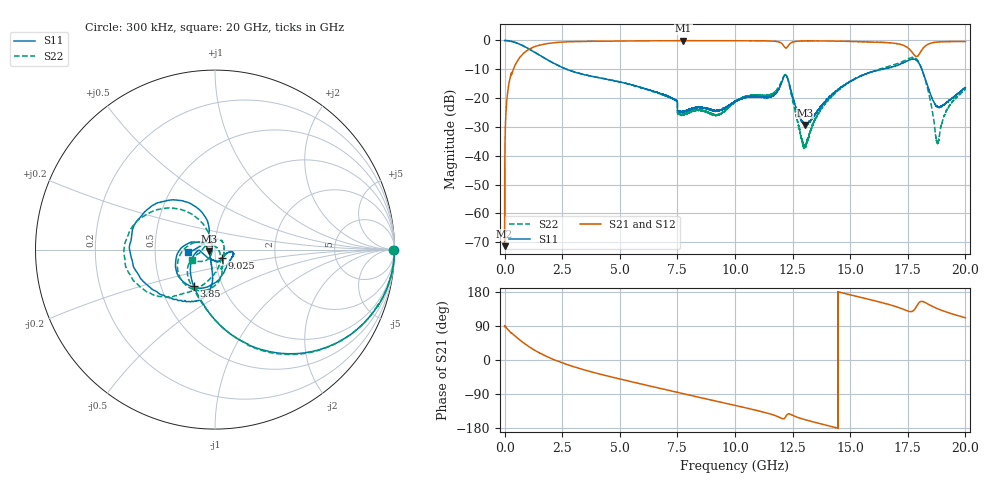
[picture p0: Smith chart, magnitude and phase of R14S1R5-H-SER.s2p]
!{R14S1R5}
!Johanson Technology Inc.
!www.johansontechnology.com
!Test Board Conditions:
!Substrate Type  RO4350B
!Substrate Thickness  20 mil
!Substrate Dk  3.66
!TL Type: GCPW
!TL Trace Width  36 mil
!TL Gap  12 mil
!Electrode orientation  Horizontal
!DUT TOPOLOGY	SERIES
!Mounting Pad LxW  26x36 mil
! Created Wed Nov 25 17:33:21 2020
! 2 Port Network Data from SP1.SP block
! freq  magS11  angS11  magS21  angS21  magS12  angS12  magS22  angS22
# khz S ma R 50
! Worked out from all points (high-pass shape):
!   20001 points, 300 kHz to 20 GHz, reference 50 ohm
!   highest |S21| = -0.06 dB at 7.757 GHz (marker M1); lowest = -71.4 dB at 300 kHz (marker M2)
!   |S21| within 3 dB of the highest: 1.064 GHz to 17.58 GHz (16.51 GHz wide, 177 % of centre); 18.13 GHz to end of sweep
!   lowest |S11| = -29.4 dB at 13.03 GHz (marker M3), VSWR 1.07, Z = 46.8 - j0.824 ohm
!   |S11| at or under -10 dB: 2.697 GHz to 16.41 GHz (13.72 GHz wide, 144 % of centre); 16.41419 GHz to 16.41645 GHz (2.262 MHz wide, 0.0138 % of centre); 18.11 GHz to end of sweep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
!   |S22| runs from -37.5 to 0.0 dB; largest |S21 - S12| = 0.015
!   S11 on the Smith chart (normalised r, x): 300 kHz: open; 3.85 GHz: 0.73, -0.31; 9.025 GHz: 1.08, -0.10; 20 GHz: 0.74, -0.02
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300  0.9959 -0.0  0.0002699 88.0  0.0002458 93.8  0.9944 -0.0
132300  0.9912 -8.6  0.126 81.2  0.1265 81.2  0.9917 -8.6
501300  0.9111 -28.7  0.4045 60.7  0.4056 60.9  0.911 -28.8
1743300  0.4912 -78.2  0.8658 11.7  0.8675 11.7  0.4915 -78.0
3334300  0.2621 -112.7  0.9603 -23.9  0.9604 -23.8  0.2636 -114.4
3850300  0.2357 -120.3  0.9664 -32.6  0.9668 -32.6  0.2367 -124.3
6667300  0.1241 -164.1  0.9873 -73.7  0.9865 -73.7  0.1215 -161.2
7757300  0.05883 -108.3  0.9932 -88.9  0.9915 -88.9  0.05241 112.3
9025300  0.06097 -50.5  0.99 -106.4  0.9919 -106.4  0.05225 17.2
1.00003e7  0.08802 -7.9  0.988 -119.8  0.9871 -119.9  0.08582 -58.4
1.16103e7  0.108 -47.2  0.9739 -144.0  0.9726 -143.9  0.1185 -70.9
1.21963e7  0.2529 -138.7  0.7407 -150.0  0.7454 -150.1  0.2556 -133.8
1.30343e7  0.03403 -165.0  0.981 -157.3  0.9802 -157.4  0.01503 39.5
1.33343e7  0.04382 -130.6  0.9828 -162.4  0.9835 -162.4  0.03103 -33.5
1.46573e7  0.1593 -95.2  0.97 177.2  0.9684 177.1  0.1547 -97.5
1.66673e7  0.3308 -120.7  0.914 146.6  0.9042 146.4  0.3569 -132.5
1.74543e7  0.4373 -156.0  0.7707 130.2  0.7655 130.1  0.4656 -153.2
1.79403e7  0.4289 145.6  0.5412 147.4  0.5414 147.9  0.4411 155.5
1.83463e7  0.1703 105.2  0.8473 148.6  0.8453 148.6  0.1541 114.5
1.87873e7  0.0708 133.8  0.9376 135.5  0.9349 135.6  0.01654 177.6
1.92343e7  0.08595 167.8  0.9538 125.4  0.9517 125.8  0.06594 -125.6
2e7  0.153 -174.3  0.9583 111.4  0.9576 111.5  0.1436 -155.4
